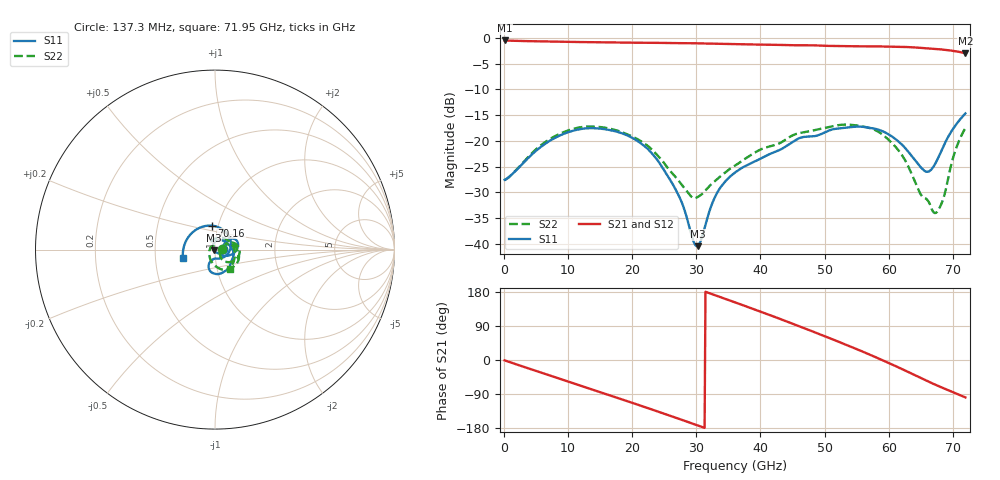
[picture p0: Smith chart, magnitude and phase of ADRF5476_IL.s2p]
! Device:  ADRF5476
! Description: Flip-Chip, Silicon Digital Step Attenuator
! Frequency:  0.1 GHz -  72 GHz
! Ports:
!  RFC = ATTIN
!  RF1 = ATTOUT
! VDD  =  +3.3 Volts
! VSS  =  -3.3 Volts
! State
! Insertion Loss State: D0 = 0V, D1 = 0V
! Data:  Data was collected using a calibrated network analyzer
!  The reference plane is the package boundry of ADRF5476 switch.
! Notes: Analog Devices supplies this data as a sample of measured data
!  for this product.  Your particular data for this product may vary.
!  Analog Devices reserves the right to change this data at anytime.
# GHZ  S  DB  R  50
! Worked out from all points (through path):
!   524 points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, 137.3 MHz to 71.95 GHz, reference 50 ohm
!   highest |S21| = -0.50 dB at 137.3 MHz (marker M1); lowest = -3.0 dB at 71.95 GHz (marker M2)
!   group delay of S21, straight-line fit = 17.5 ps
!   lowest |S11| = -40.5 dB at 30.21 GHz (marker M3), VSWR 1.02, Z = 49.2 - j0.48 ohm
!   |S11| at or under -10 dB: start of sweep to end of sweep
!   |S22| runs from -34.0 to -16.8 dB; largest |S21 - S12| = 0.026
!   S11 on the Smith chart (normalised r, x): 137.3 MHz: 1.09, +0.00; 70.16 GHz: 0.93, +0.25; 71.95 GHz: 0.69, -0.07
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0.1373092  -27.56 2.5  -0.50 -1.0  -0.50 -0.9  -27.66 2.3
5.766985  -21.19 37.0  -0.68 -32.9  -0.68 -32.9  -20.88 26.8
12.22052  -17.66 22.5  -0.81 -69.0  -0.81 -69.0  -17.31 -0.2
18.12481  -18.40 -1.1  -0.90 -102.2  -0.90 -102.2  -18.18 -30.4
21.69485  -20.78 -19.2  -0.94 -122.5  -0.93 -122.5  -20.32 -46.1
24.16641  -24.10 -33.1  -0.97 -137.0  -0.96 -137.0  -23.08 -54.2
27.32452  -30.76 -47.3  -1.02 -155.3  -1.01 -155.3  -27.86 -47.0
29.52147  -39.33 -110.2  -1.04 -168.5  -1.04 -168.4  -31.10 -21.2
30.20802  -40.45 -149.1  -1.06 -172.6  -1.06 -172.6  -30.93 -8.2
33.09151  -30.49 110.7  -1.13 170.1  -1.13 170.1  -27.64 16.3
36.11231  -26.08 80.8  -1.21 151.8  -1.20 151.8  -24.77 22.7
42.42853  -22.05 24.9  -1.35 112.5  -1.34 112.4  -20.75 15.3
48.05821  -19.13 -33.2  -1.43 75.9  -1.43 75.9  -18.02 -2.9
51.35363  -17.74 -56.1  -1.56 53.9  -1.55 53.9  -17.12 -16.4
54.78636  -17.25 -78.4  -1.63 30.3  -1.62 30.3  -16.97 -38.3
60.0041  -18.75 -106.2  -1.70 -7.9  -1.69 -8.0  -19.82 -81.2
62.33836  -21.09 -112.8  -1.75 -26.0  -1.75 -26.1  -23.30 -107.8
65.63378  -25.87 -94.3  -1.99 -52.6  -1.98 -52.7  -31.11 159.3
67.14418  -24.66 -55.8  -2.14 -64.3  -2.13 -64.2  -34.01 115.3
68.37996  -21.46 0.6  -2.27 -73.4  -2.27 -72.8  -31.69 117.6
70.16498  -17.42 97.6  -2.55 -86.0  -2.55 -84.7  -22.72 66.9
71.95  -14.66 -165.5  -2.98 -98.7  -2.98 -96.6  -17.48 -52.0
